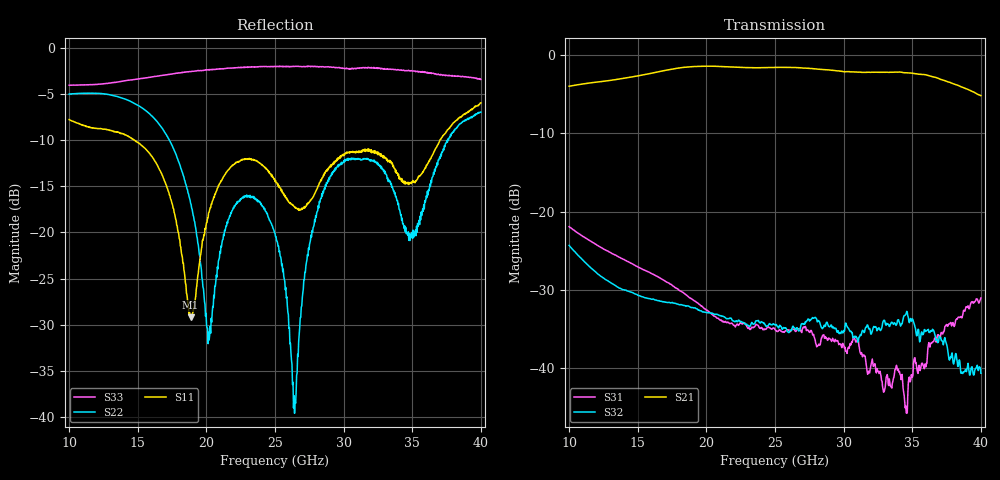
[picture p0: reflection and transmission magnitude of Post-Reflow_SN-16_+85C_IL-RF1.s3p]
!Agilent Technologies,N5245A,US49150155,A.09.90.19
!Agilent N5245A: A.09.90.19
!Date: Wednesday, November 14, 2018 03:50:46
!Correction: S11(Full 3 Port(1,2,3))
!S12(Full 3 Port(1,2,3))
!S13(Full 3 Port(1,2,3))
!S21(Full 3 Port(1,2,3))
!S22(Full 3 Port(1,2,3))
!S23(Full 3 Port(1,2,3))
!S31(Full 3 Port(1,2,3))
!S32(Full 3 Port(1,2,3))
!S33(Full 3 Port(1,2,3))
!S3P File: Measurements: <S11,S12,S13>,
!<S21,S22,S23>,
!<S31,S32,S33>:
# Hz S  dB  R 50
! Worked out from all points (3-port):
!   801 points, 10 GHz to 40 GHz, reference 50 ohm
!   strongest paths, dB at 10 GHz, 17.5 GHz, 25 GHz, 32.5 GHz, 40 GHz:
!     S21: -3.9, -1.8, -1.5, -2.2, -5.1
!     S32: -24.3, -31.7, -34.5, -35.0, -40.7
!     S31: -21.9, -29.4, -35.1, -40.5, -31.1
!   lowest |S11| = -29.2 dB at 18.85 GHz (marker M1), VSWR 1.07, Z = 46.8 - j1.12 ohm
!   |S11| at or under -10 dB: 14.73 GHz to 37.03 GHz (22.29 GHz wide, 86.1 % of centre)
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1e10  -7.80 8.3  -3.95 -159.2  -21.94 90.6
      -3.94 -159.2  -5.05 -102.6  -24.35 23.4
      -21.94 90.8  -24.33 23.6  -4.08 59.0
1.51e10  -10.36 -143.4  -2.59 92.5  -27.16 -5.6
         -2.59 92.4  -6.33 168.0  -30.78 -71.3
         -27.19 -5.3  -30.78 -71.1  -3.38 -42.7
1.885e10  -29.20 -159.9  -1.45 8.9  -31.08 -74.6
          -1.45 8.7  -16.85 98.6  -32.28 -149.3
          -31.14 -74.3  -32.26 -149.0  -2.60 -102.4
2.01625e10  -17.90 -106.2  -1.38 -21.5  -32.83 -94.8
            -1.37 -21.6  -30.81 143.0  -32.97 -177.8
            -32.81 -94.7  -32.97 -177.6  -2.43 -120.3
2.5e10  -14.50 -177.2  -1.53 -128.8  -35.11 -157.7
        -1.53 -129.0  -20.10 124.2  -34.50 73.8
        -35.14 -157.4  -34.54 74.1  -2.05 -177.6
2.6425e10  -17.25 -174.5  -1.55 -161.1  -35.22 -178.0
           -1.55 -161.3  -39.59 10.2  -34.92 44.0
           -35.19 -177.7  -34.92 44.8  -2.05 165.2
2.81875e10  -14.91 -152.7  -1.77 158.6  -36.95 153.4
            -1.76 158.5  -17.36 -113.6  -33.93 -2.9
            -36.99 153.9  -34.00 -2.7  -2.11 145.6
3.10375e10  -11.25 -179.7  -2.15 94.3  -36.50 97.6
            -2.14 94.2  -12.09 172.9  -36.71 -60.1
            -36.51 96.8  -36.75 -60.3  -2.22 109.5
3.50125e10  -14.60 161.5  -2.28 -1.5  -41.15 87.9
            -2.28 -1.6  -20.65 -4.6  -33.83 -166.1
            -41.24 89.2  -33.76 -165.9  -2.53 50.3
4e10  -5.99 122.3  -5.15 -129.8  -31.18 -14.0
      -5.15 -130.0  -7.00 139.5  -40.47 -47.8
      -31.08 -13.5  -40.72 -45.9  -3.45 -36.0
